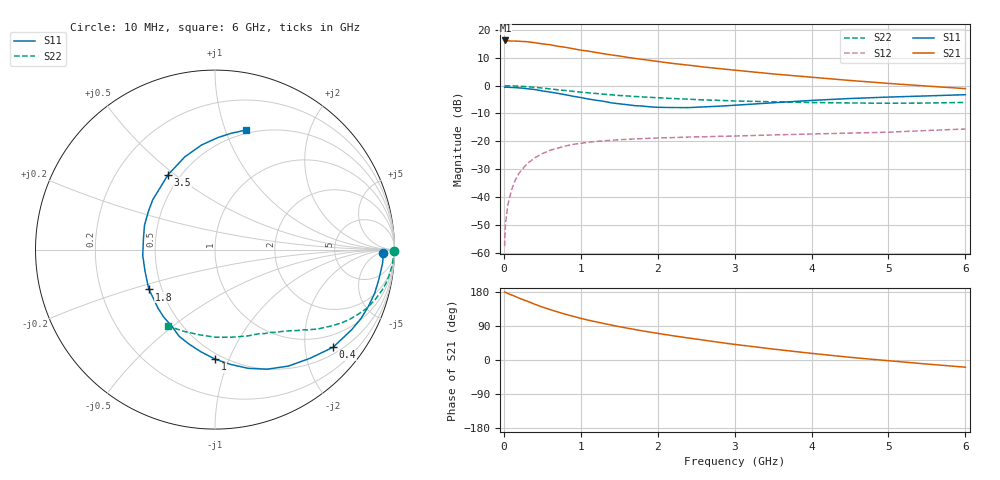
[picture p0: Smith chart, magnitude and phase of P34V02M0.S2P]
! SIEMENS Small Signal Semiconductors
! BFP181
! Si NPN RF Bipolar Junction Transistor in SOT143
! VCE = 4 V  IC = 2 mA
! Common Emitter S-Parameters:  March  1996
# GHz  S  MA  R  50
!  f  S11  S21  S12  S22
! GHz  MAG  ANG  MAG  ANG  MAG  ANG  MAG  ANG
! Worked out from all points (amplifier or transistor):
!   36 points, 10 MHz to 6 GHz, reference 50 ohm
!   highest |S21| = 16.3 dB at 20 MHz (marker M1)
!   |S21| within 3 dB of that: start of sweep to 906.2 MHz
!   unconditionally stable (mu >= 1): 2.492 GHz to end of sweep
!   at 250 MHz: K = 0.12, MSG = 22.8 dB, |S12| = -29.7 dB
!   at 1.4 GHz: K = 0.64, MSG = 15.3 dB, |S12| = -19.6 dB
!   at 6 GHz: K = 1.14, MAG = 5.0 dB, |S12| = -15.6 dB
!   lowest NFmin = 1.35 dB at 450 MHz
!   S11 on the Smith chart (normalised r, x): 10 MHz: 27, -8; 400 MHz: 0.66, -2.63; 1 GHz: 0.46, -0.89; 1.8 GHz: 0.42, -0.23; 3.5 GHz: 0.43, +0.47; 6 GHz: 0.47, +1.18
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0.01  0.9346 -1.1  6.434 179.3  0.0013 87.0  0.9969 -0.4
0.02  0.9381 -2.0  6.498 178.8  0.0031 86.6  0.9892 -0.8
0.05  0.9367 -4.8  6.419 175.8  0.007 89.4  0.9936 -2.3
0.1  0.9281 -10.2  6.341 171.7  0.0134 82.8  0.9929 -4.6
0.15  0.9223 -15.3  6.329 167.5  0.0201 80.3  0.9852 -6.9
0.25  0.8994 -25.3  6.22 159.1  0.0327 74.9  0.9697 -11.4
0.3  0.8828 -30.3  6.176 155.6  0.0392 71.8  0.9586 -13.5
0.4  0.8538 -39.6  5.923 147.3  0.0502 66.6  0.9344 -17.4
0.5  0.8041 -48.9  5.646 139.8  0.0601 61.0  0.9068 -21.1
0.6  0.7671 -57.8  5.44 133.1  0.0688 56.2  0.8752 -24.3
0.8  0.6869 -74.4  4.898 120.8  0.0821 48.3  0.8176 -29.8
1  0.6112 -89.8  4.355 110.1  0.0919 41.9  0.7648 -34.1
1.1  0.5749 -97.8  4.173 105.0  0.096 39.4  0.7426 -35.9
1.4  0.4901 -119.3  3.565 92.1  0.1044 32.7  0.6837 -40.9
1.6  0.4554 -134.2  3.245 84.2  0.1084 29.7  0.6537 -43.4
1.8  0.4299 -148.9  2.967 76.9  0.1117 27.2  0.6277 -46.0
2.2  0.404 -175.3  2.505 63.9  0.1164 23.2  0.5867 -51.1
2.8  0.4275 150.4  2.026 46.6  0.1229 19.3  0.5445 -59.2
3.5  0.4923 122.1  1.625 28.9  0.13 16.3  0.5131 -69.9
4.5  0.5873 97.4  1.24 7.1  0.1402 13.0  0.4886 -89.3
5.5  0.6541 82.1  0.983 -10.7  0.1563 11.6  0.4871 -110.5
6  0.688 75.5  0.885 -19.0  0.1662 9.6  0.4994 -121.4
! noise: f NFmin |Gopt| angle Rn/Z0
0.45  1.35  0.6  17  0.4
0.9  1.45  0.5  36  0.4
1.8  1.8  0.31  80  0.37
